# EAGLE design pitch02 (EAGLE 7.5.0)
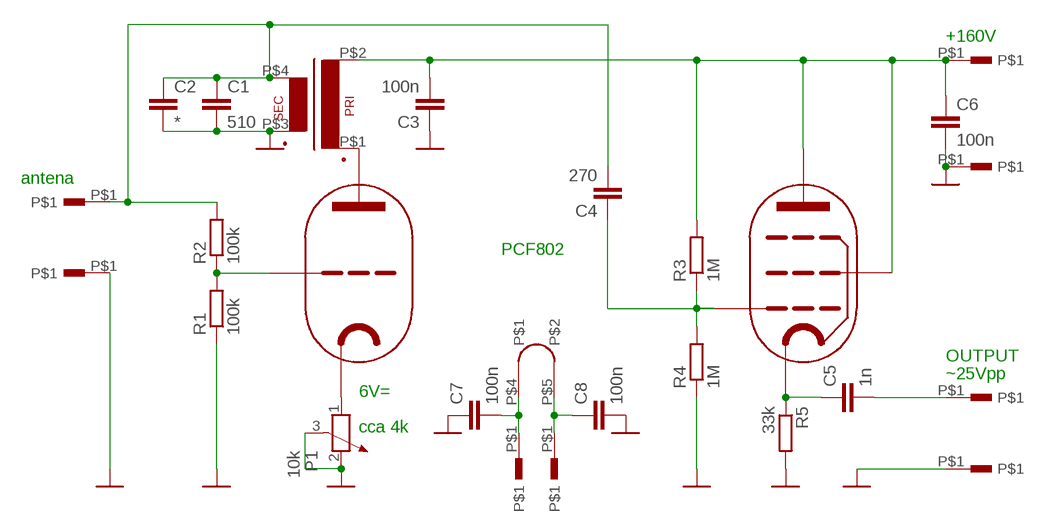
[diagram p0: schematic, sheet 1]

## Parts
C1  510  C-EU075-032X103  [C075-032X103]
C2  *  C-EU075-032X103  [C075-032X103]
C3  100n  C-EU075-032X103  [C075-032X103]
C4  270  C-EU050-024X044  [C050-024X044]
C5  1n  C-EU075-032X103  [C075-032X103]
C6  100n  C-EU075-032X103  [C075-032X103]
C7  100n  C-EU050-024X044  [C050-024X044]
C8  100n  C-EU050-024X044  [C050-024X044]
P1  10k  POTENTIOMETER_PT-10  [PT-10]
R1  100k  R-EU_0207/10  [0207/10]
R2  100k  R-EU_0207/10  [0207/10]
R3  1M  R-EU_0207/10  [0207/10]
R4  1M  R-EU_0207/10  [0207/10]
R5  33k  R-EU_0207/10  [0207/10]
U$1  PCF802  PCF82  [NOVAL02]
U$2  PIN  [PIN]
U$3  PIN  [PIN]
U$4  PIN  [PIN]
U$5  PIN  [PIN]
U$6  PIN  [PIN]
U$7  PIN  [PIN]
U$8  PIN  [PIN]
U$9  TRAFO_18  [EI18]
U$10  PIN  [PIN]

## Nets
GND: C1.2 C2.2 C3.1 C6.2 C7.1 C8.2 P1.2 P1.3 R1.1 R4.1 R5.2 U$3.P$1 U$6.P$1 U$9.P$3(S1) U$10.P$1
N$1: U$1.P$1(A) U$9.P$1(P1)
N$2: C7.2 U$1.P$4 U$7.P$1
N$3: C8.1 U$1.P$5 U$8.P$1
N$4: C5.1 R5.1 U$1.P$7(K)
N$5: C3.2 C6.1 R3.2 U$1.P$3(G2) U$1.P$6(A) U$4.P$1 U$9.P$2(P2)
N$7: R1.2 R2.1 U$1.P$9(G1)
N$9: C1.1 C2.1 C4.2 R2.2 U$2.P$1 U$9.P$4(S2)
N$12: C5.2 U$5.P$1
N$13: P1.1 U$1.P$8(K)
N$14: C4.1 R3.1 R4.2 U$1.P$2(G1)

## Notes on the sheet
- +160V
- antena
- PCF802
- OUTPUT
- ~25Vpp
- 6V=
- cca 4k

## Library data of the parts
C1-C8 = rcl:C-EU: CAPACITOR, European symbol
P1 = rcl:POTENTIOMETER_: Potentiometer
R1-R5 = rcl:R-EU_: RESISTOR, European symbol
U$1 = lampy03:PCF82
U$2-U$8 U$10 = lampy04:PIN
U$9 = trafo_ferit:TRAFO_18

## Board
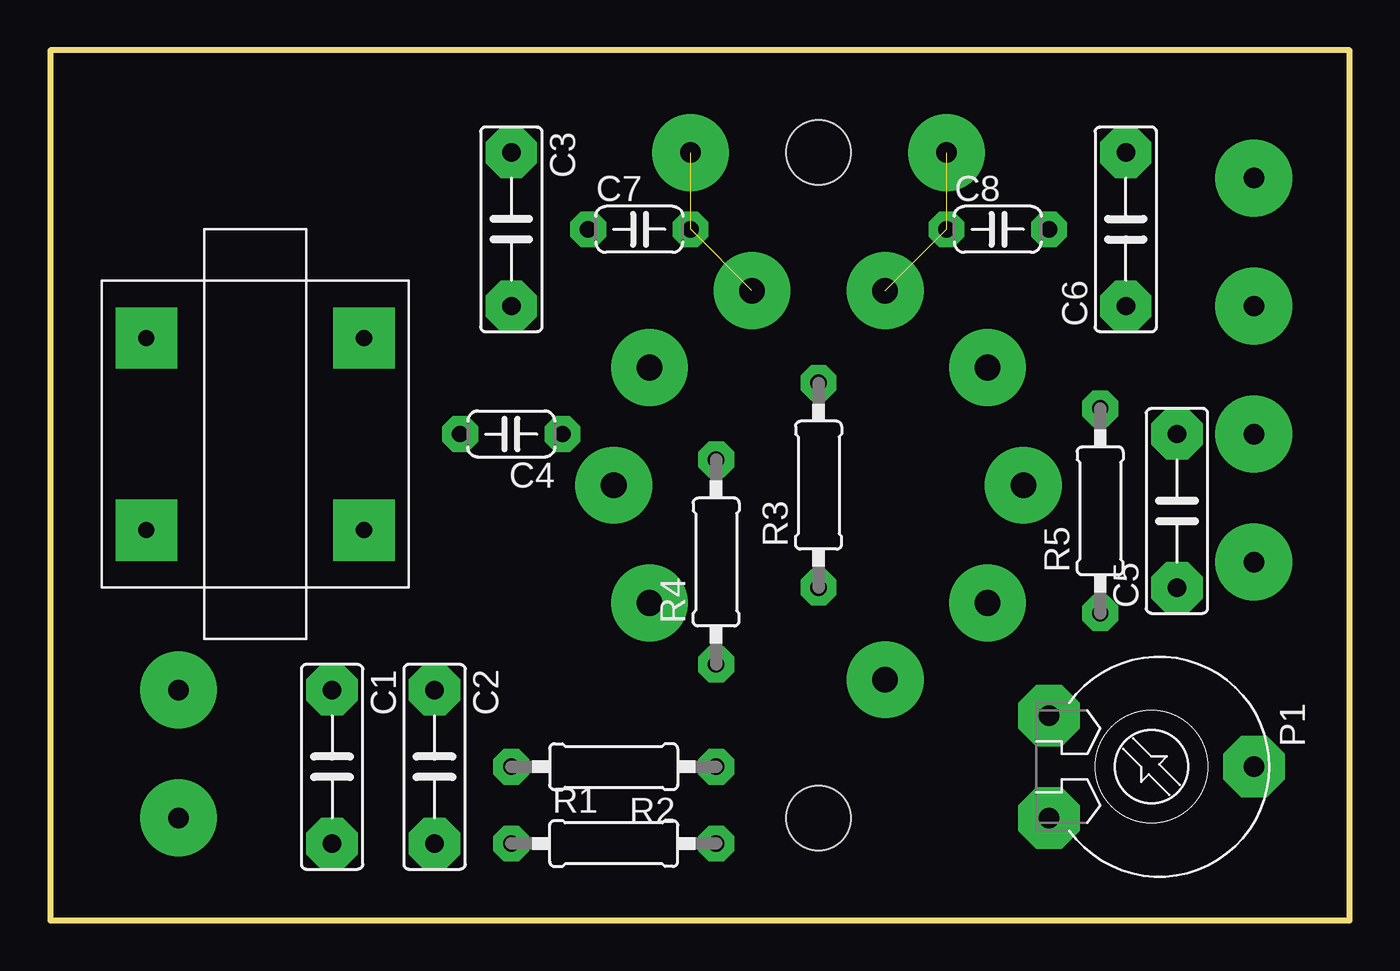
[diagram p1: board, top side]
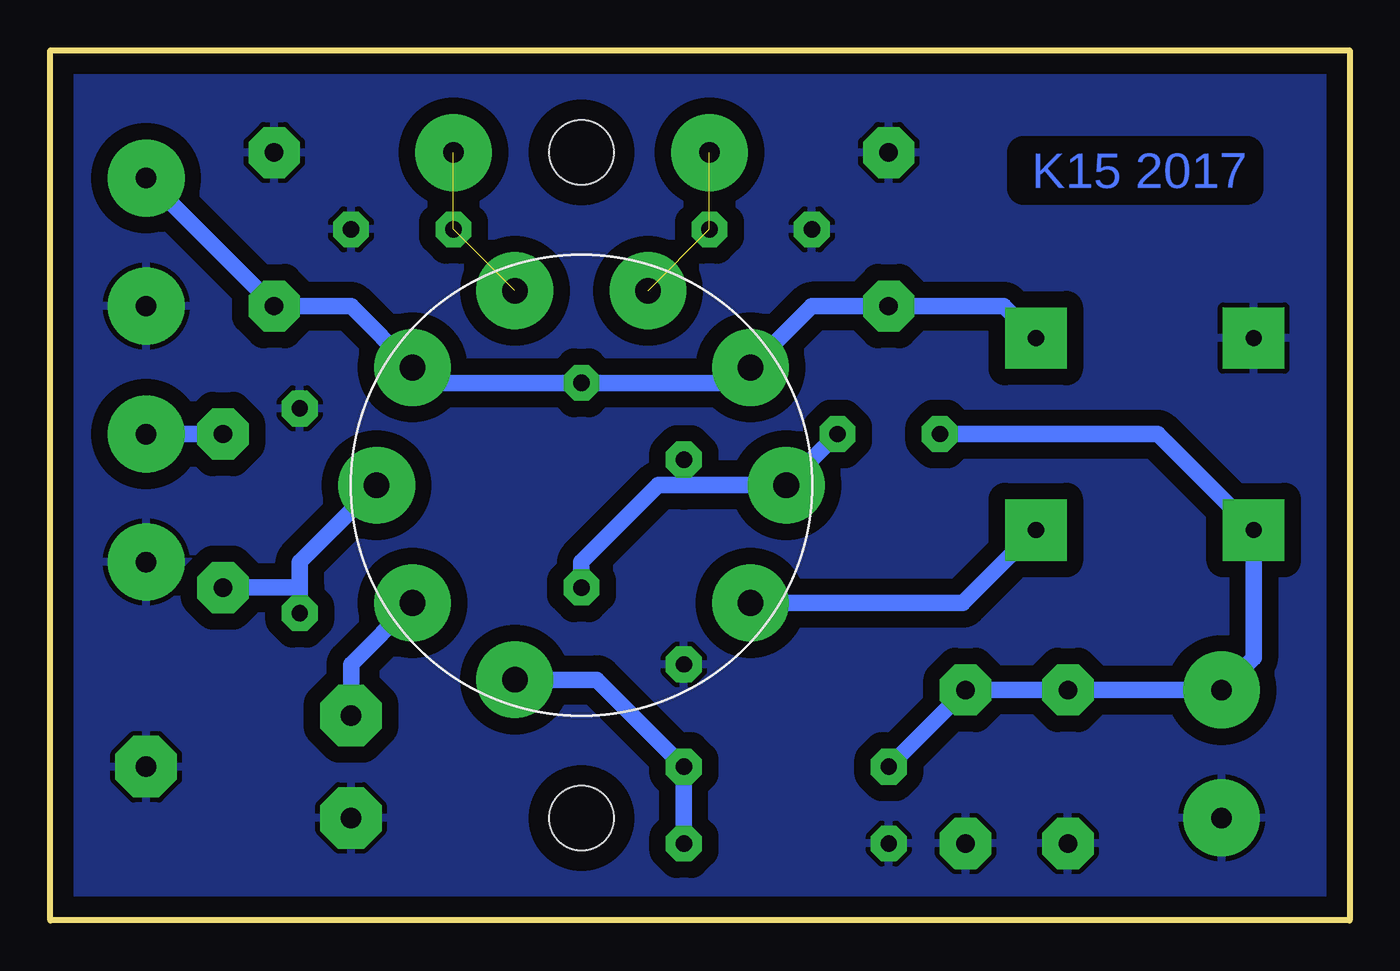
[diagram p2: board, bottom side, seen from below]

Size 64.44 x 43.17 mm. Coordinates in mm from the lower left corner, seen from the top.
Outline: 0,0 64.44,0 64.44,43.17 0,43.17 0,0
Copper layers (1*16): Top 0.035mm / dielectric 1.5mm / Bottom 0.035mm
Design rules "default": minimum track width 10mil, minimum drill 24mil, track to track 8mil, track to pad 8mil, pad to pad 8mil, via to via 8mil, smd to smd 8mil, copper to edge 40mil, drill to drill 8mil, minimum pad ring 10mil, minimum via ring 8mil, stop-mask expansion 4mil, vias tented up to drill 0mil, thermal gap 10mil
Holes 3.2 mm at 38.1,38.1 38.1,5.08

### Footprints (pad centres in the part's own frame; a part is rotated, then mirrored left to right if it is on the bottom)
C075-032X103 = drill 0.914 pad 2.54 octagon: 1 -3.81,0; 2 3.81,0
C050-024X044 = drill 0.813 pad 1.778 octagon: 1 -2.54,0; 2 2.54,0
PT-10 = drill 1.016 pad 3.048 octagon: 1 -2.54,-5.08; 2 2.54,-5.08; 3 0,5.08
0207/10 = drill 0.813 pad 1.778 octagon: 1 -5.08,0; 2 5.08,0
NOVAL02 = drill 1.27 pad 3.81: P$1 8.382,-5.842; P$2 10.16,0; P$3 8.382,5.842; P$4 3.302,9.652; P$5 -3.302,9.652; P$6 -8.382,5.842; P$7 -10.16,0; P$8 -8.382,-5.842; P$9 -3.302,-9.652
PIN = drill 1.016 pad 3.81: P$1 0,0
EI18 = drill 0.8 pad 3.048 square: P$1 -4.763,-5.397; P$2 4.763,-5.397; P$3 4.763,5.397; P$4 -4.763,5.397

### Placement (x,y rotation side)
C1  13.97,7.62 270 top
C2  19.05,7.62 270 top
C3  22.86,34.29 270 top
C4  22.86,24.13 180 top
C5  55.88,20.32 90 top
C6  53.34,34.29 90 top
C7  29.21,34.29 0 top
C8  46.99,34.29 0 top
P1  54.61,7.62 270 top
R1  27.94,3.81 0 top
R2  27.94,7.62 180 top
R3  38.1,21.59 90 top
R4  33.02,17.78 90 top
R5  52.07,20.32 90 top
U$1  38.1,21.59 0 bottom
U$2  6.35,11.43 0 top
U$3  6.35,5.08 0 top
U$4  59.69,36.83 0 top
U$5  59.69,24.13 0 top
U$6  59.69,17.78 0 top
U$7  31.75,38.1 0 top
U$8  44.45,38.1 0 top
U$9  10.16,24.13 90 top
U$10  59.69,30.48 0 top

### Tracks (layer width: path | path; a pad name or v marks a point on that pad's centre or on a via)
GND
  pour Bottom (isolate 0.813): 0,43.18 64.77,43.18 64.77,0 0,0
N$1
  Bottom 0.813: U$1.P$1 19.18,15.75 U$9.P$1
N$2  (2 unrouted)
N$3  (2 unrouted)
N$4
  Bottom 0.813: C5.1 52.07,16.51 R5.1 52.07,17.78 U$1.P$7
N$5
  Bottom 0.813: U$4.P$1 C6.1 49.53,30.48 U$1.P$6 45.72,26.67 R3.2 30.48,26.67 U$1.P$3 26.67,30.48 C3.2 17.14,30.48 U$9.P$2
N$7
  Bottom 0.813: U$1.P$9 37.34,11.94 R2.1 R1.2
N$9
  Bottom 0.813: R2.2 C2.1 C1.1 U$2.P$1 4.76,13.02 U$9.P$4 9.53,24.13 C4.2
N$12
  Bottom 0.813: U$5.P$1 C5.2
N$13
  Bottom 0.813: P1.1 49.53,12.7 U$1.P$8
N$14
  Bottom 0.813: 33.02,21.59 U$1.P$2 C4.1 | 33.02,21.59 34.29,21.59 38.1,17.78 R3.1 | R4.2 33.02,21.59

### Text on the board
Bottom: K15 2017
